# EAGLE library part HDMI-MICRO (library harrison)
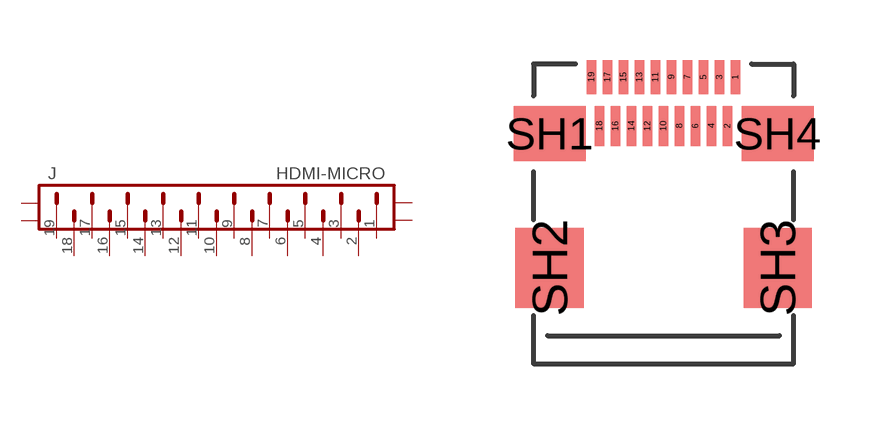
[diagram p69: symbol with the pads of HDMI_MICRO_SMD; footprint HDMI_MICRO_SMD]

Designator prefix J

## HDMI-MICRO  [HDMI_MICRO_SMD]
1  1  pas
2  2  pas
3  3  pas
4  4  pas
5  5  pas
6  6  pas
7  7  pas
8  8  pas
9  9  pas
10  10  pas
11  11  pas
12  12  pas
13  13  pas
14  14  pas
15  15  pas
16  16  pas
17  17  pas
18  18  pas
19  19  pas
SH1  SH1  pas
SH2  SH2  pas
SH3  SH3  pas
SH4  SH4  pas

## Footprint HDMI_MICRO_SMD (pad centres in mm)
smd 0.23 x 0.85: 1 1.8,3.475; 3 1.4,3.475; 5 1,3.475; 7 0.6,3.475; 9 0.2,3.475; 11 -0.2,3.475; 13 -0.6,3.475; 15 -1,3.475; 17 -1.4,3.475; 19 -1.8,3.475
smd 0.23 x 1: 2 1.6,2.25; 4 1.2,2.25; 6 0.8,2.25; 8 0.4,2.25; 10 0,2.25; 12 -0.4,2.25; 14 -0.8,2.25; 16 -1.2,2.25; 18 -1.6,2.25
smd 1.8 x 1.38: SH1 -2.85,2.06; SH4 2.85,2.06
smd 1.7 x 2: SH2 -2.85,-1.3; SH3 2.85,-1.3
